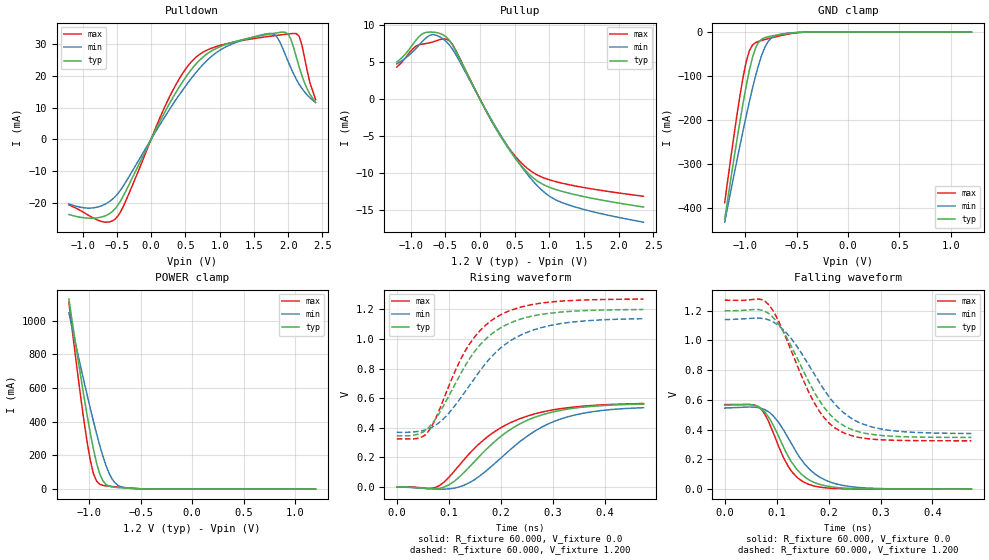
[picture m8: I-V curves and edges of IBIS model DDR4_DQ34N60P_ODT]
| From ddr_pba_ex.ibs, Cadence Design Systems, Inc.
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|   Model DDR4_DQ34N60P_ODT
[Model]   DDR4_DQ34N60P_ODT
Model_type I/O
Polarity   Non-Inverting
Enable   Active-High
Vinl   =  823550V
Vinh   =  887750V
C_comp   1.703pF   1.712pF   1.718pF
C_comp_pullup   0.536pF   0.593pF   0.524pF
C_comp_pulldown 1.166pF   1.119pF   1.193pF
[Model Spec]
Vinh   0.887V   NA   NA
Vinl   0.823V   NA   NA
Vmeas   0.840V   NA   NA
[Add Submodel]
|  Submodel_name   Mode
DDR4_DQ_ODT60   Non-Driving
[Temperature Range]   27.000   0.125k   -40.000
[Voltage Range]   1.200V   1.140V   1.270V
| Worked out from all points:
|   slope of the pulldown table from 0 to 0.18 V, typ, clamps not added: 23.3 ohm
|   slope of the pullup table from 0 to 0.18 V, typ, clamps not added: 57.4 ohm
|   GND clamp passes 1 mA (typ) near -0.50 V on its own axis
|   POWER clamp passes 1 mA (typ) near -0.46 V on its own axis
|   rising waveform, R_fixture 60.000, V_fixture 0.0: 20-80 % time 116ps typ, 122ps min, 118ps max; typ from 0.001 V to 0.56 V
|   rising waveform, R_fixture 60.000, V_fixture 1.200: 20-80 % time 95.8ps typ, 111ps min, 86.1ps max; typ from 0.346 V to 1.2 V
|   falling waveform, R_fixture 60.000, V_fixture 0.0: 20-80 % time 54.2ps typ, 65.2ps min, 45.8ps max; typ from 0.565 V to 0 V
|   falling waveform, R_fixture 60.000, V_fixture 1.200: 20-80 % time 80.7ps typ, 90.9ps min, 74.1ps max; typ from 1.2 V to 0.348 V
[Pulldown]
|Voltage   I(typ)   I(min)   I(max)
-1.2V     -23.72mA   -20.38mA   -20.68mA
-840mV    -24.88mA   -21.61mA   -24.88mA
-520mV    -21.78mA   -18mA      -25.05mA
400mV     16.1mA     13.66mA    18.67mA
640mV     23.35mA    20.64mA    25.58mA
960mV     28.73mA    27.44mA    29.28mA
1.76V     33.27mA    33.33mA    32.54mA
1.84V     33.56mA    32.14mA    32.76mA
2V        33.13mA    24.48mA    33.18mA
2.12V     25.82mA    18.86mA    33.28mA
2.2V      20.09mA    16.05mA    29.74mA
2.4V      11.64mA    11.56mA    12.48mA
[Pullup]
|Voltage   I(typ)   I(min)   I(max)
-1.2V     5.02mA     4.773mA    4.338mA
-960mV    7.516mA    6.485mA    6.876mA
-840mV    8.783mA    7.706mA    7.425mA
-720mV    9.066mA    8.641mA    7.63mA
-560mV    8.818mA    8.321mA    8.099mA
-400mV    7.394mA    6.807mA    7.432mA
280mV     -4.745mA   -4.576mA   -4.71mA
520mV     -8.111mA   -8.075mA   -7.827mA
760mV     -10.57mA   -11.01mA   -9.882mA
960mV     -11.75mA   -12.82mA   -10.77mA
1.2V      -12.51mA   -14.04mA   -11.39mA
2.36V     -14.59mA   -16.63mA   -13.13mA
[GND_clamp]
|Voltage   I(typ)   I(min)   I(max)
-1.2V     -426.2mA   -432.8mA   -388.3mA
-1.08V    -244.1mA   -290.9mA   -187.6mA
-1.02V    -160.2mA   -222.9mA   -101.2mA
-990mV    -121.8mA   -190.1mA   -66.76mA
-960mV    -87.12mA   -158.5mA   -42.47mA
-900mV    -36.37mA   -100.2mA   -23.99mA
-840mV    -16.17mA   -52.6mA    -18.98mA
-810mV    -12.75mA   -34.94mA   -17.06mA
-750mV    -9.219mA   -14.09mA   -13.42mA
-600mV    -3.476mA   -2.979mA   -5.372mA
-390mV    -77.95uA   -145.6uA   -88.64uA
1.2V      1.573nA    185.8nA    251.5pA
[POWER_clamp]
|Voltage   I(typ)   I(min)   I(max)
-1.2V     1.129A     1.047A     1.109A
-1.08V    651.1mA    713.3mA    524.8mA
-1.02V    430.1mA    553.1mA    270.8mA
-990mV    328mA      475.7mA    167mA
-960mV    234.7mA    400.6mA    90.32mA
-930mV    154.2mA    328.7mA    47.17mA
-900mV    91.53mA    260.8mA    29.3mA
-840mV    28.2mA     142.5mA    19.67mA
-780mV    13.3mA     60.49mA    15.94mA
-720mV    9.309mA    21.57mA    12.7mA
-660mV    6.902mA    8.818mA    9.642mA
1.2V      -4.11nA    -153.5nA   -872pA
[Ramp]
| variable   typ   min   max
dV/dt_r 0.301/0.113n   0.290/0.120n   0.299/0.111n
dV/dt_f 0.481/82.284p   0.430/94.734p   0.535/76.742p
R_load = 50.000
| The next line is not an IBIS keyword
| [Initial Delay]   0.325ns   0.520ns   0.200ns
[Rising Waveform]
R_fixture= 60.000
V_fixture= 0.0
V_fixture_min= 0.0
V_fixture_max= 0.0
|time   V(typ)   V(min)   V(max)
0s        1.472mV    660.6uV    338.7uV
66ps      -11.39mV   -11.28mV   -9.106mV
99ps      12.2mV     -12.89mV   61.27mV
138ps     129.2mV    25.84mV    218.9mV
170ps     246.7mV    103mV      326.5mV
213ps     375.2mV    235.5mV    424.8mV
249ps     447.3mV    338mV      476.5mV
286ps     493.9mV    417.1mV    511.1mV
336ps     529.9mV    481mV      538.3mV
475ps     560.2mV    535.7mV    563.9mV
[Rising Waveform]
R_fixture= 60.000
V_fixture= 1.200
V_fixture_min= 1.140
V_fixture_max= 1.270
|time   V(typ)   V(min)   V(max)
0s        346.1mV    369.6mV    325.1mV
37ps      353.4mV    373.4mV    326.6mV
58ps      391.2mV    388.8mV    363.3mV
89ps      542.9mV    457.3mV    583.1mV
134ps     832.4mV    655.4mV    932.3mV
160ps     958.8mV    784.1mV    1.055V
199ps     1.072V     936.2mV    1.161V
238ps     1.133V     1.025V     1.214V
296ps     1.174V     1.091V     1.249V
475ps     1.198V     1.137V     1.269V
[Falling Waveform]
R_fixture= 60.000
V_fixture= 0.0
V_fixture_min= 0.0
V_fixture_max= 0.0
|time   V(typ)   V(min)   V(max)
0s        564.6mV    545.3mV    569mV
54ps      565.8mV    552.1mV    567.4mV
71ps      538.5mV    542.6mV    534.5mV
94ps      425.4mV    490.5mV    375mV
122ps     223.1mV    345mV      154.1mV
137ps     140.9mV    254.4mV    88.68mV
161ps     65.71mV    142.2mV    33.27mV
196ps     21.33mV    57.53mV    8.435mV
245ps     4.537mV    15.89mV    1.576mV
475ps     107.8uV    117.5uV    48.05uV
[Falling Waveform]
R_fixture= 60.000
V_fixture= 1.200
V_fixture_min= 1.140
V_fixture_max= 1.270
|time   V(typ)   V(min)   V(max)
0s        1.199V     1.14V      1.27V
65ps      1.208V     1.15V      1.278V
84ps      1.182V     1.139V     1.243V
123ps     995.7mV    1.034V     974.7mV
170ps     668.2mV    787mV      595.7mV
191ps     551.5mV    670.7mV    481.8mV
218ps     453mV      550.1mV    399mV
256ps     387.8mV    452.5mV    349.5mV
295ps     363.2mV    408.7mV    333.1mV
475ps     347.6mV    374mV      325.1mV
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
